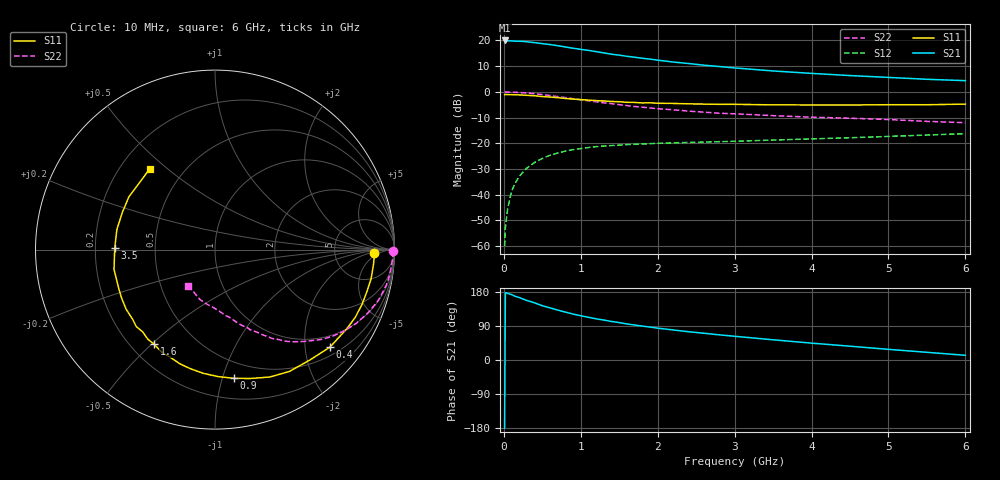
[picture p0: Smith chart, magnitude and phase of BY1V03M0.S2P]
! SIEMENS Small Signal Semiconductors
! BFY420
! Si NPN RF SIEGET Grounded Emitter Transistor in MICRO-X
! VCE = 1 V  IC = 3 mA
! Common Emitter S-Parameters:  October  1996
# GHz  S  MA  R  50
!  f  S11  S21  S12  S22
! GHz  MAG  ANG  MAG  ANG  MAG  ANG  MAG  ANG
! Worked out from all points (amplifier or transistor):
!   36 points, 10 MHz to 6 GHz, reference 50 ohm
!   highest |S21| = 20.0 dB at 10 MHz (marker M1)
!   |S21| within 3 dB of that: start of sweep to 896.2 MHz
!   unconditionally stable (mu >= 1): 3.554 GHz to end of sweep
!   at 250 MHz: K = 0.08, MSG = 25.4 dB, |S12| = -31.2 dB
!   at 1.4 GHz: K = 0.41, MSG = 17.8 dB, |S12| = -20.9 dB
!   at 6 GHz: K = 1.21, MAG = 7.5 dB, |S12| = -16.3 dB
!   S11 on the Smith chart (normalised r, x): 10 MHz: 16, -3; 400 MHz: 0.70, -2.57; 900 MHz: 0.36, -1.09; 1.6 GHz: 0.29, -0.51; 3.5 GHz: 0.28, +0.01; 6 GHz: 0.32, +0.43
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0.01  0.8881 -1.1  10.01 -179.7  0.001 94.0  0.9923 -0.6
0.02  0.8883 -2.2  9.992 178.1  0.0023 88.4  0.9901 -1.1
0.05  0.8869 -5.3  9.784 175.6  0.0054 87.1  0.9914 -2.9
0.1  0.8848 -10.6  9.805 172.7  0.0117 84.5  0.9865 -5.9
0.15  0.878 -15.6  9.673 167.8  0.0171 80.9  0.9815 -8.9
0.2  0.8738 -20.8  9.651 164.9  0.0226 78.4  0.975 -11.7
0.25  0.8676 -25.9  9.594 160.8  0.0277 74.7  0.9628 -14.7
0.4  0.8403 -40.2  9.081 150.8  0.0425 67.3  0.9213 -22.7
0.5  0.8109 -49.4  8.667 143.2  0.0509 62.6  0.8869 -27.7
0.6  0.7954 -58.6  8.33 137.6  0.0585 58.3  0.8494 -32.4
0.7  0.7729 -66.7  7.915 131.8  0.0647 54.2  0.8118 -36.6
0.9  0.7246 -81.8  7.068 121.2  0.0754 46.5  0.7375 -43.5
1.1  0.6921 -95.6  6.411 112.7  0.0829 41.2  0.6715 -49.9
1.4  0.6508 -112.1  5.403 101.7  0.0906 34.6  0.5905 -57.1
1.6  0.6271 -122.7  4.924 95.1  0.0945 31.5  0.5413 -61.0
2  0.6013 -139.6  4.145 84.0  0.0999 26.7  0.4706 -67.5
2.2  0.5963 -146.1  3.811 79.3  0.1021 24.9  0.4491 -70.4
2.8  0.5729 -163.9  3.116 66.4  0.1077 21.6  0.385 -78.1
3.5  0.5588 179.2  2.555 53.3  0.1158 19.1  0.3453 -85.8
4.5  0.5562 158.2  2.076 36.4  0.1284 15.8  0.3077 -98.3
5.5  0.5624 138.1  1.758 20.3  0.145 12.0  0.2672 -115.4
6  0.5784 129.1  1.654 12.4  0.1539 9.7  0.2523 -126.0
